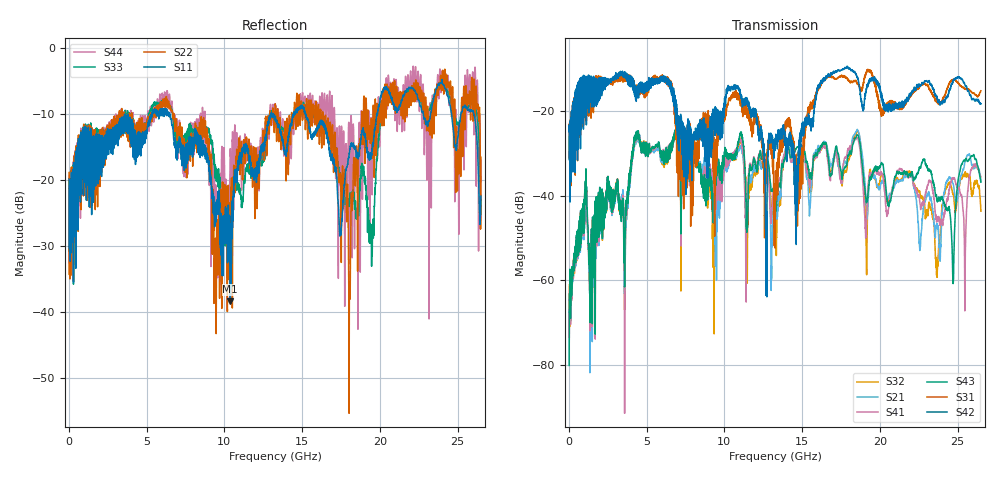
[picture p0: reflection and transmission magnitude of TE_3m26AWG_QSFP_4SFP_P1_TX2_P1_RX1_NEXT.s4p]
!Agilent Technologies,N5222A,MY51421691,A.10.00.00
!Agilent N5222A: A.10.00.00
!Date: Friday, January 30, 2015 12:33:53
!Correction: S11(Full 4 Port(1,2,3,4))
!S12(Full 4 Port(1,2,3,4))
!S13(Full 4 Port(1,2,3,4))
!S14(Full 4 Port(1,2,3,4))
!S21(Full 4 Port(1,2,3,4))
!S22(Full 4 Port(1,2,3,4))
!S23(Full 4 Port(1,2,3,4))
!S24(Full 4 Port(1,2,3,4))
!S31(Full 4 Port(1,2,3,4))
!S32(Full 4 Port(1,2,3,4))
!S33(Full 4 Port(1,2,3,4))
!S34(Full 4 Port(1,2,3,4))
!S41(Full 4 Port(1,2,3,4))
!S42(Full 4 Port(1,2,3,4))
!S43(Full 4 Port(1,2,3,4))
!S44(Full 4 Port(1,2,3,4))
!S4P File: Measurements: <S11,S12,S13,S14>,
!<S21,S22,S23,S24>,
!<S31,S32,S33,S34>,
!<S41,S42,S43,S44>:
# Hz S  dB  R 50.0
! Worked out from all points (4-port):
!   2650 points, 10 MHz to 26.5 GHz, reference 50 ohm
!   strongest paths, dB at 10 MHz, 6.63 GHz, 13.26 GHz, 19.88 GHz, 26.5 GHz:
!     S42: -24.9, -16.1, -29.4, -13.2, -18.3
!     S31: -24.7, -15.5, -42.5, -17.3, -15.3
!     S43: -80.1, -28.5, -39.8, -33.6, -36.9
!     S41: -67.9, -28.1, -37.9, -34.5, -35.6
!     S21: -72.2, -28.2, -40.1, -38.1, -36.6
!     S32: -69.5, -28.6, -43.4, -38.1, -43.7
!   lowest |S11| = -38.3 dB at 10.38 GHz (marker M1), VSWR 1.02, Z = 49.1 + j0.771 ohm
!   |S11| at or under -10 dB: start of sweep to 3.58 GHz; 6.485 GHz to 12.98 GHz (6.494 GHz wide, 66.7 % of centre); 15.24 GHz to 19.8 GHz (4.556 GHz wide, 26 % of centre)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
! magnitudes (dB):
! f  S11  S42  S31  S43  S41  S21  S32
! 10 MHz  -19.8  -24.9  -24.7  -80.1  -67.9  -72.2  -69.5
! 1.03 GHz  -11.8  -12.3  -13.3  -40.9  -41.5  -42.0  -41.4
! 4.35 GHz  -16.1  -14.8  -14.6  -25.2  -25.5  -25.7  -25.4
! 10.38 GHz  -38.3  -15.1  -17.6  -31.0  -31.4  -31.4  -31.4
! 12.68 GHz  -13.0  -45.2  -37.1  -30.4  -31.7  -31.9  -30.8
! 17.24 GHz  -20.2  -10.8  -12.4  -29.0  -30.8  -30.8  -29.9
! 26.5 GHz  -22.4  -18.3  -15.3  -36.9  -35.6  -36.6  -43.7
